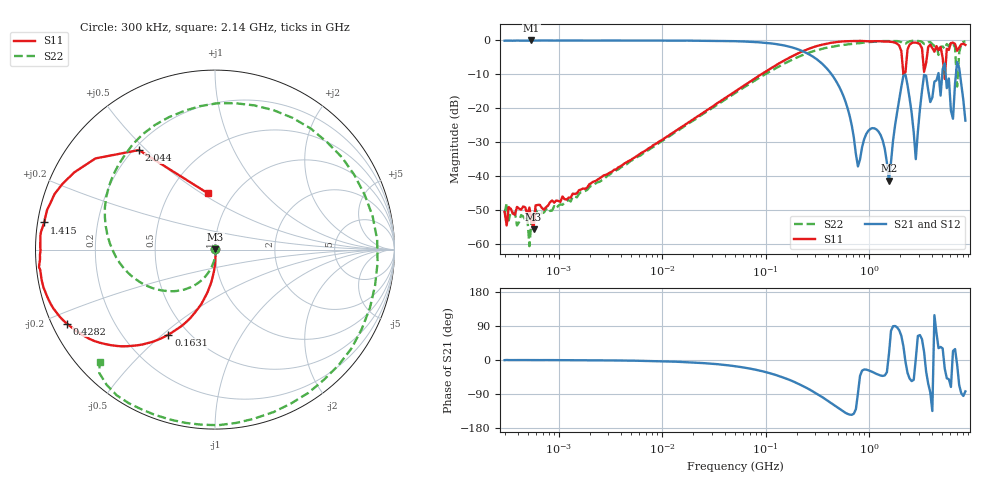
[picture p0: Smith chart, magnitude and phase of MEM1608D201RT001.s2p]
! S-Parameter Data Generated by TDK Corporation
! Copyright(C) 2025 TDK Corporation.
! All Rights Reserved.
! TDK P/N: MEM1608D201RT001 (3-terminal Filter)
! Property: Fc=200MHz
! Size(LxWxT): 1.6x0.8x0.6mm
! Model Type: s2p (Touchstone File Format Version 1.0)
! Frequency: DC=Yes Start=0.3MHz Stop=8500MHz 225points Log-sweep
! Model Generated on Feb. 6, 2025
! Terms and conditions regarding TDK Simulation Models:
! 1)This simulation model is being provided solely for informational
!  purposes. Please refer to the specifications of the products in
!  terms of detailed characteristics of such products.
! 2)In no event shall TDK Corporation of any of its subsidiaries be
!  liable for any loss or damage arising, directly or indirectly,
!  from any information contained in this simulation model, including,
!  but not limited to loss or damages arising from any inaccuracies,
!  omissions or errors in connection with such information.
! 3)Any and all copyrights on this simulation model are owned by
!  TDK Corporation.  Duplication or redistribution of this simulation
!  model without prior written permission from TDK Corporation
!  is prohibited.
! 4)This simulation model is subject to any modification or change
!  without any prior notice.
! 5)Neither TDK Corporation nor any of its subsidiaries shall make any
!  warranty, express or implied, including but not limited to the
!  correctness, implied warranties of merchantability and fitness for
!  a particular purpose with respect to this simulation models.
! 6)The use of this simulation model shall be deemed to have consented
!  to the terms and conditions hereof.
! Port Assignments:
!  1 ---@@@--- 2
! Applicable Conditions:
!  Temperature = 25 degC
!  DC Bias Current = 0 A
!  DC Bias Voltage = 0 V
!  Small Signal Operation
# Hz S MA R 50
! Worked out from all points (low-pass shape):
!   224 points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, 300 kHz to 8.5 GHz, reference 50 ohm
!   highest |S21| = 0.00 dB at 545.3 kHz (marker M1); lowest = -41.3 dB at 1.551 GHz (marker M2)
!   |S21| within 3 dB of the highest: start of sweep to 221.1 MHz
!   lowest |S11| = -55.6 dB at 571 kHz (marker M3), VSWR 1.00, Z = 50.1 + j0.125 ohm
!   |S11| at or under -10 dB: start of sweep to 90.19 MHz; 5.316 GHz to 5.405 GHz (89.07 MHz wide, 1.66 % of centre)
!   |S22| runs from -60.6 to -0.1 dB; largest |S21 - S12| = 0.023
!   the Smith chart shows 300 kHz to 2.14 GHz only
!   S11 on the Smith chart (normalised r, x): 300 kHz: 1.00, +0.01; 163.1 MHz: 0.39, -0.52; 428.2 MHz: 0.04, -0.24; 1.415 GHz: 0.02, +0.08; 2.044 GHz: 0.22, +0.48; 2.14 GHz: 0.76, +0.53
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300000  0.002981 68.5  0.9911 -0.4  0.9917 0.0  0.002897 82.8
545346.1  0.002226 107.8  1 -0.3  1 1.1  0.002226 73.0
571002.1  0.001656 48.7  0.9956 -0.5  0.9995 -1.0  0.002606 44.0
1721110  0.006586 -47.7  0.997 -0.6  0.9948 -0.6  0.005866 -56.2
9430415  0.0327 -83.6  0.9955 -3.1  0.9943 -3.0  0.03121 -87.1
5.167171e7  0.1818 -96.4  0.9746 -16.7  0.974 -16.6  0.1714 -111.4
1.630757e8  0.5409 -118.7  0.8209 -50.6  0.82 -50.4  0.484 -161.7
2.831228e8  0.7897 -137.7  0.5843 -82.5  0.5821 -82.2  0.6883 149.2
4.282171e8  0.9231 -153.5  0.3243 -113.7  0.3243 -113.4  0.8036 95.9
7.784218e8  0.9802 -173.4  0.01396 -88.0  0.01396 -88.1  0.9087 -4.6
1.415031e9  0.9633 171.0  0.02522 -40.7  0.0254 -40.4  0.9784 -94.4
1.551304e9  0.9613 166.6  0.008562 15.4  0.008616 15.5  0.9794 -104.9
2.044041e9  0.6981 127.4  0.2076 63.8  0.2081 63.9  0.9424 -133.2
2.140204e9  0.3167 97.3  0.3035 36.2  0.3051 36.3  0.896 -135.8
2.346313e9  0.7363 -150.0  0.2194 -34.2  0.2208 -34.1  0.9426 -136.6
2.819992e9  0.9292 167.4  0.01784 3.1  0.01788 3.0  0.9887 -150.8
3.389298e9  0.3457 96.8  0.3111 21.8  0.3113 21.9  0.8879 -163.9
3.548748e9  0.4663 -136.1  0.3025 -30.8  0.3024 -30.4  0.8917 -161.2
5.367404e9  0.2713 -120.6  0.4608 -22.6  0.4603 -22.3  0.753 -172.4
6.450987e9  0.929 157.2  0.07028 23.8  0.07103 24.5  0.9069 157.9
7.072242e9  0.7055 143.7  0.4802 -12.4  0.4827 -11.8  0.2097 122.0
8.5e9  0.8596 124.6  0.06591 -82.9  0.06572 -82.3  0.9731 175.7
